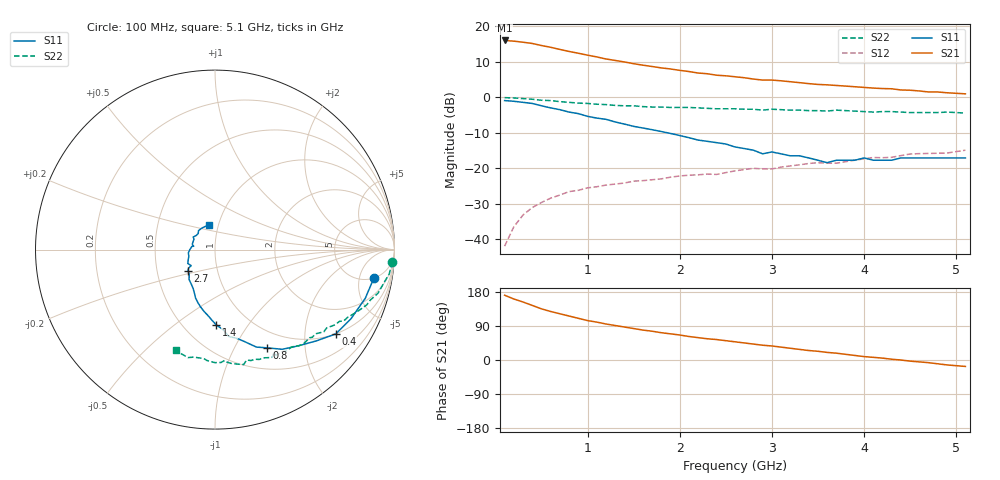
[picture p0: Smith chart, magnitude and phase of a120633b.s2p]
!  INA-12063 S PARAMETERS
!  Vd = 3 V  Id = 2.5 mA  LAST UPDATED 10-07-96
# ghz s ma r 50
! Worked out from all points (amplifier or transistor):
!   51 points, 100 MHz to 5.1 GHz, reference 50 ohm
!   highest |S21| = 16.0 dB at 100 MHz (marker M1)
!   |S21| within 3 dB of that: start of sweep to 782.4 MHz
!   unconditionally stable (mu >= 1): 1.283 GHz to end of sweep
!   at 900 MHz: K = 0.72, MSG = 19.3 dB, |S12| = -26.2 dB
!   at 2.6 GHz: K = 1.48, MAG = 9.2 dB, |S12| = -20.7 dB
!   at 5.1 GHz: K = 1.57, MAG = 3.5 dB, |S12| = -14.9 dB
!   S11 on the Smith chart (normalised r, x): 100 MHz: 5.09, -8.37; 400 MHz: 1.00, -2.86; 800 MHz: 0.77, -1.36; 1.4 GHz: 0.71, -0.72; 2.7 GHz: 0.72, -0.18; 5.1 GHz: 0.91, +0.25
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0.1  0.9 -10.0  6.33 171.0  0.008 87.0  0.99 -4.0
0.2  0.88 -18.0  6.19 161.0  0.015 79.0  0.98 -8.0
0.3  0.85 -27.0  5.98 153.0  0.022 73.0  0.96 -11.0
0.4  0.82 -35.0  5.74 144.0  0.028 68.0  0.94 -15.0
0.5  0.76 -42.0  5.37 135.0  0.033 62.0  0.91 -18.0
0.6  0.71 -49.0  5.07 128.0  0.038 59.0  0.9 -20.0
0.8  0.62 -62.0  4.43 116.0  0.047 53.0  0.85 -25.0
1  0.54 -72.0  3.93 104.0  0.053 49.0  0.82 -29.0
1.2  0.49 -81.0  3.47 95.0  0.058 46.0  0.79 -32.0
1.4  0.42 -89.0  3.15 87.0  0.062 44.0  0.76 -35.0
1.6  0.37 -96.0  2.84 79.0  0.067 41.0  0.74 -39.0
1.8  0.33 -104.0  2.6 72.0  0.071 41.0  0.73 -42.0
2.1  0.27 -115.0  2.31 62.0  0.08 38.0  0.72 -47.0
2.2  0.25 -119.0  2.2 59.0  0.081 36.0  0.71 -49.0
2.6  0.2 -136.0  1.95 48.0  0.092 36.0  0.69 -55.0
2.7  0.19 -142.0  1.89 45.0  0.096 35.0  0.68 -57.0
2.9  0.16 -146.0  1.75 39.0  0.098 29.0  0.66 -60.0
3.1  0.16 -159.0  1.71 34.0  0.104 33.0  0.67 -64.0
3.5  0.13 172.0  1.52 23.0  0.12 25.0  0.65 -72.0
4  0.14 150.0  1.38 9.0  0.136 25.0  0.63 -84.0
4.3  0.13 136.0  1.32 2.0  0.143 21.0  0.63 -90.0
5.1  0.14 103.0  1.12 -17.0  0.18 10.0  0.6 -111.0
